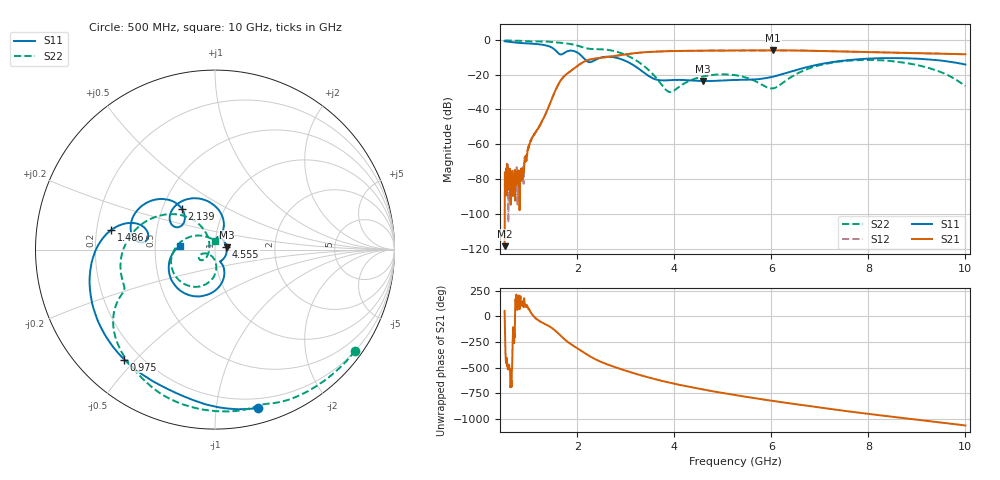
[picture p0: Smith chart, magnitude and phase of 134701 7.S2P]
!  2-Port S-parameters saved by WinCal
! VAR MeasName=S-Parameters (CALIBRATED_DATA) read from VNA (N5242A)
! VAR MeasDate=2013-7-3 16:23:31
! VAR NAME=134701 7
! VAR FILENAME=134701 7.S2P
! VAR DATE=2013-7-3 16:23:31
! VAR PHYS_PORTS=1,2
# Hz S MA R 50
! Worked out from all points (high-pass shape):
!   1601 points, 500 MHz to 10 GHz, reference 50 ohm
!   highest |S21| = -6.02 dB at 6.04 GHz (marker M1); lowest = -118.6 dB at 500 MHz (marker M2)
!   |S21| within 3 dB of the highest: 2.825 GHz to end of sweep
!   lowest |S11| = -23.7 dB at 4.585 GHz (marker M3), VSWR 1.14, Z = 56.9 + j1.41 ohm
!   |S11| at or under -10 dB: 2.115 GHz to 2.508 GHz (393.6 MHz wide, 17 % of centre); 2.76 GHz to end of sweep
!   |S22| runs from -30.1 to -0.3 dB; largest |S21 - S12| = 0.0024
!   S11 on the Smith chart (normalised r, x): 500 MHz: 0.12, -1.30; 975 MHz: 0.14, -0.46; 1.486 GHz: 0.26, +0.09; 2.139 GHz: 0.63, +0.31; 4.555 GHz: 1.14, +0.04; 10 GHz: 0.67, +0.03
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5e8  0.9145 -74.7  1.175e-06 53.8  6.945e-05 -95.5  0.9632 -35.9
8.503125e8  0.8099 -116.0  0.0001256 134.2  0.0001659 90.3  0.9371 -60.9
9.75e8  0.7943 -129.6  0.0007116 92.8  0.000661 85.5  0.9127 -69.7
1.26e9  0.733 -161.8  0.004255 -56.4  0.004283 -57.8  0.9013 -88.7
1.485625e9  0.5883 169.3  0.02215 -117.7  0.0221 -117.7  0.8709 -105.8
1.699375e9  0.3951 173.7  0.08203 151.5  0.08183 151.3  0.8133 -122.2
1.865625e9  0.492 159.6  0.1289 88.6  0.1281 88.6  0.7582 -135.2
2.085312e9  0.3487 130.5  0.215 21.3  0.2141 21.3  0.6293 -150.9
2.13875e9  0.2915 129.0  0.2367 4.9  0.2359 4.9  0.5967 -153.2
2.394062e9  0.2759 150.2  0.2947 -64.6  0.2938 -64.6  0.5432 -161.5
2.649375e9  0.3289 128.0  0.326 -115.0  0.325 -114.9  0.5111 180.0
3.142188e9  0.1932 78.4  0.4099 167.6  0.4097 167.7  0.294 138.0
3.670625e9  0.07011 76.9  0.4654 97.9  0.4647 97.9  0.06741 122.2
3.925938e9  0.06972 77.4  0.476 69.1  0.4759 69.1  0.0318 177.6
4.555312e9  0.06616 14.5  0.4894 8.0  0.4892 8.0  0.08651 -138.5
4.585e9  0.06558 10.9  0.4894 5.4  0.4892 5.5  0.08861 -139.1
5.25e9  0.07024 -54.3  0.4958 -49.0  0.4959 -49.0  0.09692 -156.3
6.039688e9  0.08783 -64.3  0.5002 -106.9  0.4996 -106.9  0.04062 -119.5
6.835312e9  0.1776 -75.7  0.4873 -161.1  0.4879 -161.1  0.1616 -94.7
8.420625e9  0.2999 -132.4  0.4337 103.1  0.4325 103.1  0.2501 -167.6
9.329062e9  0.2675 -163.2  0.4071 51.6  0.4082 51.6  0.1428 148.2
1e10  0.1957 173.7  0.3856 14.0  0.3855 13.9  0.04736 88.1
